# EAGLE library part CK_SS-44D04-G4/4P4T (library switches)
Through hole 4P4T switch.
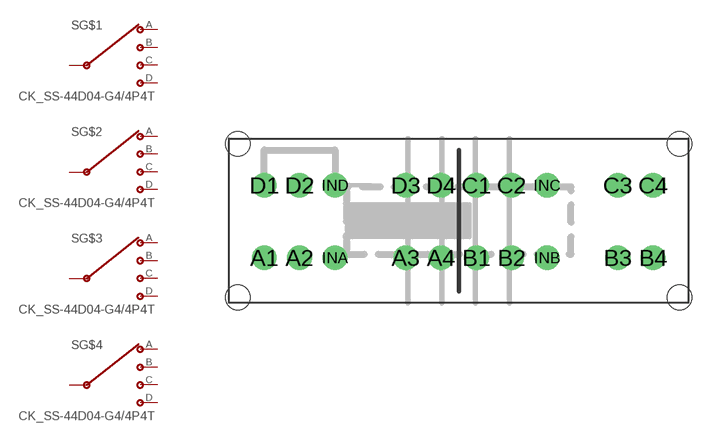
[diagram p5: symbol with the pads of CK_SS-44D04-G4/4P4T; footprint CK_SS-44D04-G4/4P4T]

Designator prefix S; gates G$1=SP4T G$2=SP4T G$3=SP4T G$4=SP4T

## CK_SS-44D04-G4/4P4T  [CK_SS-44D04-G4/4P4T]
A1  G$1:A
A2  G$1:B
A3  G$1:C
A4  G$1:D
B1  G$2:A
B2  G$2:B
B3  G$2:C
B4  G$2:D
C1  G$3:A
C2  G$3:B
C3  G$3:C
C4  G$3:D
D1  G$4:A
D2  G$4:B
D3  G$4:C
D4  G$4:D
INA  G$1:INPUT
INB  G$2:INPUT
INC  G$3:INPUT
IND  G$4:INPUT

## Footprint CK_SS-44D04-G4/4P4T (pad centres in mm)
4P4T
drill 0.8 pad 1.4: A1 -11,-2.1; A2 -9,-2.1; A3 -3,-2.1; A4 -1,-2.1; B1 1,-2.1; B2 3,-2.1; B3 9,-2.1; B4 11,-2.1; C1 1,2; C2 3,2; C3 9,2; C4 11,2; D1 -11,2; D2 -9,2; D3 -3,2; D4 -1,2; INA -7,-2.1; INB 5,-2.1; INC 5,2; IND -7,2
hole 1.4 at -12.5,4.35
hole 1.4 at 12.5,4.35
hole 1.4 at -12.5,-4.35
hole 1.4 at 12.5,-4.35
